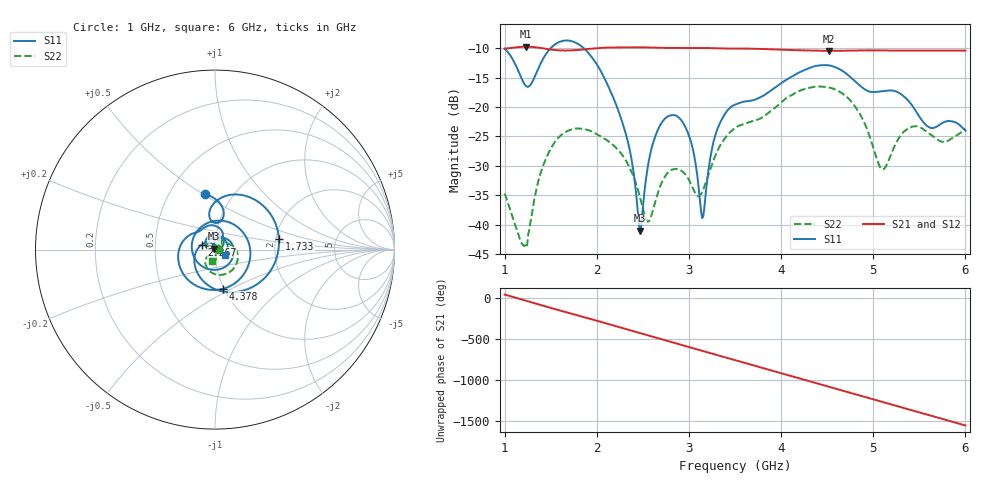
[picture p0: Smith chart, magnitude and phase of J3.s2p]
!Agilent Technologies,E8364B,MY43040528,A.07.50.67
!Agilent E8364B: A.07.50.67
!Date: Sunday, March 01, 2026 18:58:32
!Correction: S11(Full 2 Port(1,2))
!S21(Full 2 Port(1,2))
!S12(Full 2 Port(1,2))
!S22(Full 2 Port(1,2))
!S2P File: Measurements: S11, S21, S12, S22:
# Hz S  dB  R 50
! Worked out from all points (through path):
!   451 points, 1 GHz to 6 GHz, reference 50 ohm
!   highest |S21| = -9.75 dB at 1.233 GHz (marker M1); lowest = -10.5 dB at 4.522 GHz (marker M2)
!   group delay of S21, straight-line fit = 890 ps
!   lowest |S11| = -41.0 dB at 2.467 GHz (marker M3), VSWR 1.02, Z = 49.3 + j0.588 ohm
!   |S11| at or under -10 dB: start of sweep to 1.499 GHz; 1.859 GHz to end of sweep
!   |S22| runs from -43.7 to -16.5 dB; largest |S21 - S12| = 0.0015
!   S11 on the Smith chart (normalised r, x): 1 GHz: 0.74, +0.51; 1.733 GHz: 2.08, +0.29; 2.267 GHz: 0.86, +0.05; 4.378 GHz: 0.99, -0.45; 6 GHz: 1.12, -0.07
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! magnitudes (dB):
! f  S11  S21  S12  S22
! 1 GHz  -10.1  -10.1  -10.1  -34.7
! 1.233 GHz  -16.4  -9.7  -9.8  -43.1
! 1.433 GHz  -11.4  -10.1  -10.1  -29.4
! 1.733 GHz  -8.8  -10.4  -10.4  -23.8
! 1.844 GHz  -9.8  -10.2  -10.3  -23.7
! 2.267 GHz  -22.1  -9.9  -9.9  -28.0
! 2.378 GHz  -29.0  -9.9  -9.9  -31.1
! 2.467 GHz  -41.0  -9.9  -9.9  -35.2
! 2.556 GHz  -30.0  -9.9  -9.9  -39.5
! 2.667 GHz  -23.8  -9.9  -10.0  -34.5
! 2.956 GHz  -23.3  -10.0  -10.0  -31.4
! 3.144 GHz  -38.9  -10.0  -10.0  -34.5
! 3.289 GHz  -24.7  -10.0  -10.1  -28.2
! 3.5 GHz  -19.6  -10.1  -10.1  -23.6
! 4.344 GHz  -13.2  -10.4  -10.4  -16.6
! 4.378 GHz  -13.0  -10.4  -10.5  -16.5
! 4.522 GHz  -12.9  -10.5  -10.5  -16.7
! 4.833 GHz  -16.1  -10.4  -10.4  -20.6
! 5.078 GHz  -17.4  -10.4  -10.4  -30.3
! 5.167 GHz  -17.2  -10.4  -10.4  -29.1
! 5.4 GHz  -19.3  -10.4  -10.4  -23.5
! 6 GHz  -24.0  -10.4  -10.5  -23.7
